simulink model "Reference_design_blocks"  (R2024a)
settings: Solver=VariableStepAuto  StartTime=0.0  StopTime=10.0  RelTol=1e-3
libraries: matrix_library x6, dspsrcs4 x3, aieUtilities x2

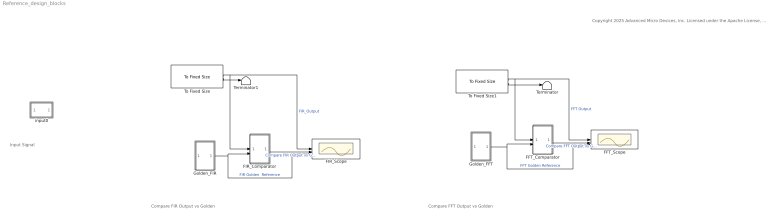
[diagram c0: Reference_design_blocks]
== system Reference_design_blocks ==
  note: Input Signal
  note: Compare FIR Output vs Golden
  note: Compare FFT Output vs Golden
  note: Copyright 2025 Advanced Micro Devices, Inc. Licensed under the Apache License, Version 2.0 (the "License"); you may not use this file except in compliance with the License. You may obtain a copy of the License at http://www.apache.org/licenses/LICENSE-2.0 Unless required by applicable law or agreed to in writing, software distributed under the License is distributed on an "AS IS" BASIS, WITHOUT WARRANTIES OR CONDITIONS OF ANY KIND, either express or implied. See the License for the specific language governing permissions and limitations under the License.
  FFT_Comparator : Subsystem
  FFT_Scope : Scope  NumInputPorts=3
  FIR_Comparator : Subsystem
  FIR_Scope : Scope  NumInputPorts=3
  Golden_FFT : Subsystem
  Golden_FIR : Subsystem
  Terminator : Terminator
  Terminator1 : Terminator
  To Fixed Size : aieUtilities/To Fixed Size  Mode=Produce a valid output signal  OutputSize=2048  CopyMethod=Buffer samples to form output  HasStatusOutput=on
  To Fixed Size1 : aieUtilities/To Fixed Size  Mode=Produce a valid output signal  OutputSize=2048  CopyMethod=Buffer samples to form output  HasStatusOutput=on
  input0 : Subsystem
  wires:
  Golden_FIR/1(Out1) -> FIR_Scope/3, FIR_Comparator/2(In2)  "FIR Golden  Reference"
  FFT_Comparator/1(Out1) -> FFT_Scope/2  "Compare FFT Output vs Golden Reference"
  Golden_FFT/1(Out1) -> FFT_Scope/3, FFT_Comparator/2(In2)  "FFT Golden Reference"
  To Fixed Size1/1 -> FFT_Scope/1, FFT_Comparator/1(In1)  "FFT Output"
  FIR_Comparator/1(Out1) -> FIR_Scope/2  "Compare FIR Output vs Golden"
  To Fixed Size/2 -> Terminator1/1
  To Fixed Size/1 -> FIR_Scope/1, FIR_Comparator/1(In1)  "FIR_Output"
  To Fixed Size1/2 -> Terminator/1

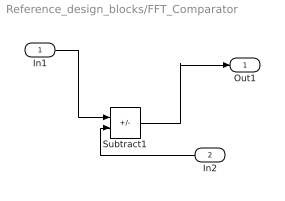
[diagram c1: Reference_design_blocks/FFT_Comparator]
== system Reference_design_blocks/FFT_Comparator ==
  In1 : Inport
  In2 : Inport  Port=2
  Subtract1 : Sum  Inputs=+-  OutDataTypeStr=double
  Out1 : Outport
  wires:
  In1/1 -> Subtract1/1
  In2/1 -> Subtract1/2
  Subtract1/1 -> Out1/1

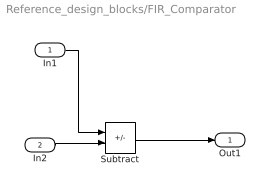
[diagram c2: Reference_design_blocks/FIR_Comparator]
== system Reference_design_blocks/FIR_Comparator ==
  In1 : Inport
  In2 : Inport  Port=2
  Subtract : Sum  Inputs=+-
  Out1 : Outport
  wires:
  Subtract/1 -> Out1/1
  In2/1 -> Subtract/2
  In1/1 -> Subtract/1

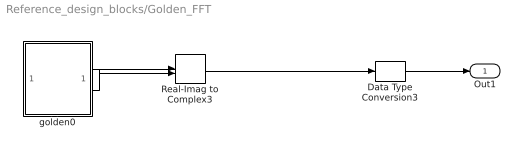
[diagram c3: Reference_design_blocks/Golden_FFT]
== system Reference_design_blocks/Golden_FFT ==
  Data Type Conversion3 : DataTypeConversion  OutDataTypeStr=int16
  Real-Imag to Complex3 : RealImagToComplex
  golden0 : Subsystem
  Out1 : Outport
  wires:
  Real-Imag to Complex3/1 -> Data Type Conversion3/1
  golden0/2(Out2) -> Real-Imag to Complex3/2
  golden0/1(Out1) -> Real-Imag to Complex3/1
  Data Type Conversion3/1 -> Out1/1

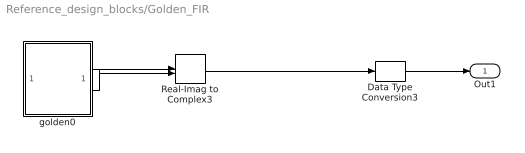
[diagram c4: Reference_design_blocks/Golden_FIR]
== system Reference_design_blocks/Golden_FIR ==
  Data Type Conversion3 : DataTypeConversion  OutDataTypeStr=int16
  Real-Imag to Complex3 : RealImagToComplex
  golden0 : Subsystem
  Out1 : Outport
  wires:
  Real-Imag to Complex3/1 -> Data Type Conversion3/1
  golden0/2(Out2) -> Real-Imag to Complex3/2
  golden0/1(Out1) -> Real-Imag to Complex3/1
  Data Type Conversion3/1 -> Out1/1

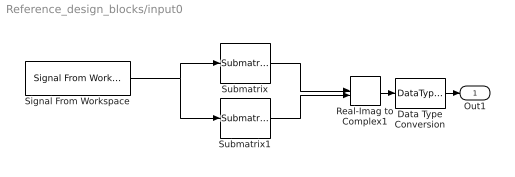
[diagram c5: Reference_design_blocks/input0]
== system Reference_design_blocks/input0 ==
  Data Type Conversion : DataTypeConversion  OutDataTypeStr=int16
  Real-Imag to Complex1 : RealImagToComplex
  Signal From Workspace : dspsrcs4/Signal From Workspace  X=PreprocIndata  Ts=1  nsamps=2048  OutputAfterFinalValue=Setting to zero  ignoreOrWarnInputAndFrameLengths=off  OutputFrames=off
  Submatrix : matrix_library/Submatrix  RowSpan=All rows  RowStartMode=First  RowStartIndex=1  RowEndMode=Last  RowEndIndex=1  ColSpan=One column  ColStartMode=First  ColStartIndex=1  ColEndMode=Last  ColEndIndex=1
  Submatrix1 : matrix_library/Submatrix  RowSpan=All rows  RowStartMode=First  RowStartIndex=1  RowEndMode=Last  RowEndIndex=1  ColSpan=One column  ColStartMode=Last  ColStartIndex=1  ColEndMode=Last  ColEndIndex=1
  Out1 : Outport
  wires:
  Signal From Workspace/1 -> Submatrix1/1, Submatrix/1
  Submatrix/1 -> Real-Imag to Complex1/1
  Submatrix1/1 -> Real-Imag to Complex1/2
  Real-Imag to Complex1/1 -> Data Type Conversion/1
  Data Type Conversion/1 -> Out1/1

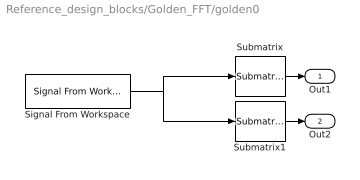
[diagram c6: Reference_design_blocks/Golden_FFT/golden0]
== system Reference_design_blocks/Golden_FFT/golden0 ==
  Signal From Workspace : dspsrcs4/Signal From Workspace  X=PreprocFftOutdata  Ts=1  nsamps=2048  OutputAfterFinalValue=Setting to zero  ignoreOrWarnInputAndFrameLengths=on  OutputFrames=off
  Submatrix : matrix_library/Submatrix  RowSpan=All rows  RowStartMode=First  RowStartIndex=1  RowEndMode=Last  RowEndIndex=1  ColSpan=One column  ColStartMode=First  ColStartIndex=1  ColEndMode=Last  ColEndIndex=1
  Submatrix1 : matrix_library/Submatrix  RowSpan=All rows  RowStartMode=First  RowStartIndex=1  RowEndMode=Last  RowEndIndex=1  ColSpan=One column  ColStartMode=Last  ColStartIndex=1  ColEndMode=Last  ColEndIndex=1
  Out1 : Outport  VectorParamsAs1DForOutWhenUnconnected=off
  Out2 : Outport  Port=2  VectorParamsAs1DForOutWhenUnconnected=off
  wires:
  Submatrix/1 -> Out1/1
  Signal From Workspace/1 -> Submatrix/1, Submatrix1/1
  Submatrix1/1 -> Out2/1

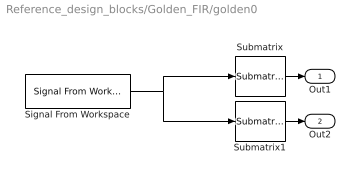
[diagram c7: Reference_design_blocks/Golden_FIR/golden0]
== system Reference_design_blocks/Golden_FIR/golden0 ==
  Signal From Workspace : dspsrcs4/Signal From Workspace  X=PreprocFirOutdata  Ts=1  nsamps=2048  OutputAfterFinalValue=Setting to zero  ignoreOrWarnInputAndFrameLengths=on  OutputFrames=off
  Submatrix : matrix_library/Submatrix  RowSpan=All rows  RowStartMode=First  RowStartIndex=1  RowEndMode=Last  RowEndIndex=1  ColSpan=One column  ColStartMode=First  ColStartIndex=1  ColEndMode=Last  ColEndIndex=1
  Submatrix1 : matrix_library/Submatrix  RowSpan=All rows  RowStartMode=First  RowStartIndex=1  RowEndMode=Last  RowEndIndex=1  ColSpan=One column  ColStartMode=Last  ColStartIndex=1  ColEndMode=Last  ColEndIndex=1
  Out1 : Outport  VectorParamsAs1DForOutWhenUnconnected=off
  Out2 : Outport  Port=2  VectorParamsAs1DForOutWhenUnconnected=off
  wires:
  Submatrix/1 -> Out1/1
  Signal From Workspace/1 -> Submatrix/1, Submatrix1/1
  Submatrix1/1 -> Out2/1
